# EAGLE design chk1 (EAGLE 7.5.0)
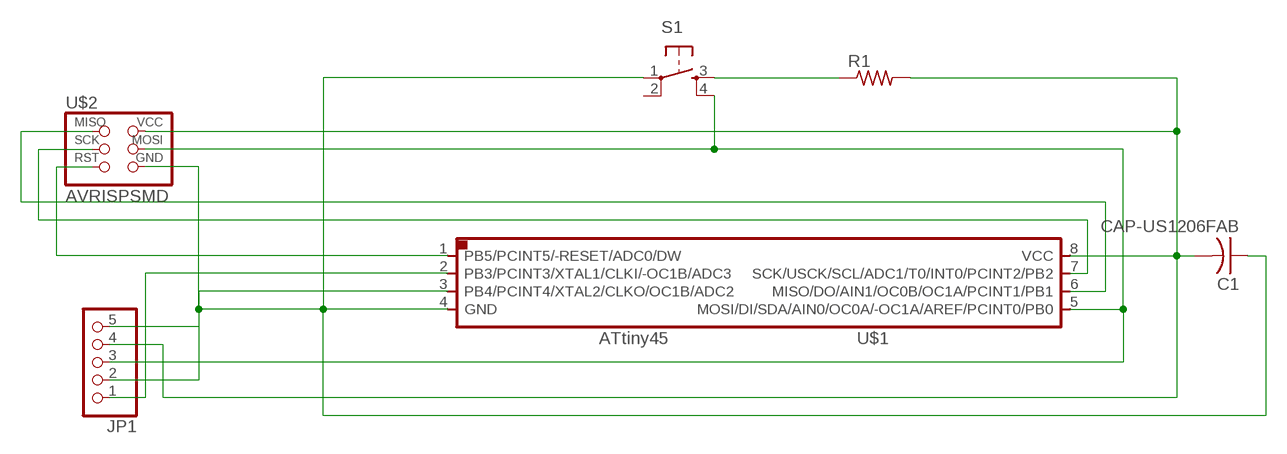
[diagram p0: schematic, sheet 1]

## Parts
C1  CAP-US1206FAB  [C1206FAB]
JP1  PINHD-1X5  [1X05]
R1  RES-US1206FAB  [R1206FAB]
S1  6MM_SWITCH6MM_SWITCH  [6MM_SWITCH]
U$1  ATTINY45SI  [SOIC8]
U$2  AVRISPSMD  [2X03SMD]

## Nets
N$1: C1.1 JP1.5 S1.1(P) U$1.4(GND) U$2.6(GND)
N$2: C1.2 JP1.4 R1.2 U$1.8(VCC) U$2.2(VCC)
N$3: U$1.6(MISO/DO/AIN1/OC0B/OC1A/PCINT1/PB1) U$2.1(MISO)
N$4: U$1.7(SCK/USCK/SCL/ADC1/T0/INT0/PCINT2/PB2) U$2.3(SCK)
N$5: JP1.3 S1.4(S1) U$1.5(MOSI/DI/SDA/AIN0/OC0A/-OC1A/AREF/PCINT0/PB0) U$2.4(MOSI)
N$6: U$1.1(PB5/PCINT5/-RESET/ADC0/DW) U$2.5(RST)
N$7: JP1.2 U$1.3(PB4/PCINT4/XTAL2/CLKO/OC1B/ADC2)
N$8: JP1.1 U$1.2(PB3/PCINT3/XTAL1/CLKI/-OC1B/ADC3)
N$9: R1.1 S1.3(S)
Unconnected: S1.2(P1)

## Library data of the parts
C1 = fab:CAP-US
JP1 = pinhead:PINHD-1X5: PIN HEADER
R1 = fab:RES-US: Resistor (US Symbol)
S1 = fab:6MM_SWITCH: OMRON SWITCH
U$1 = fab:ATTINY45
U$2 = fab:AVRISP

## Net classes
0 default: width 0.406 mm, drill 0.406 mm, clearance 0.406 mm

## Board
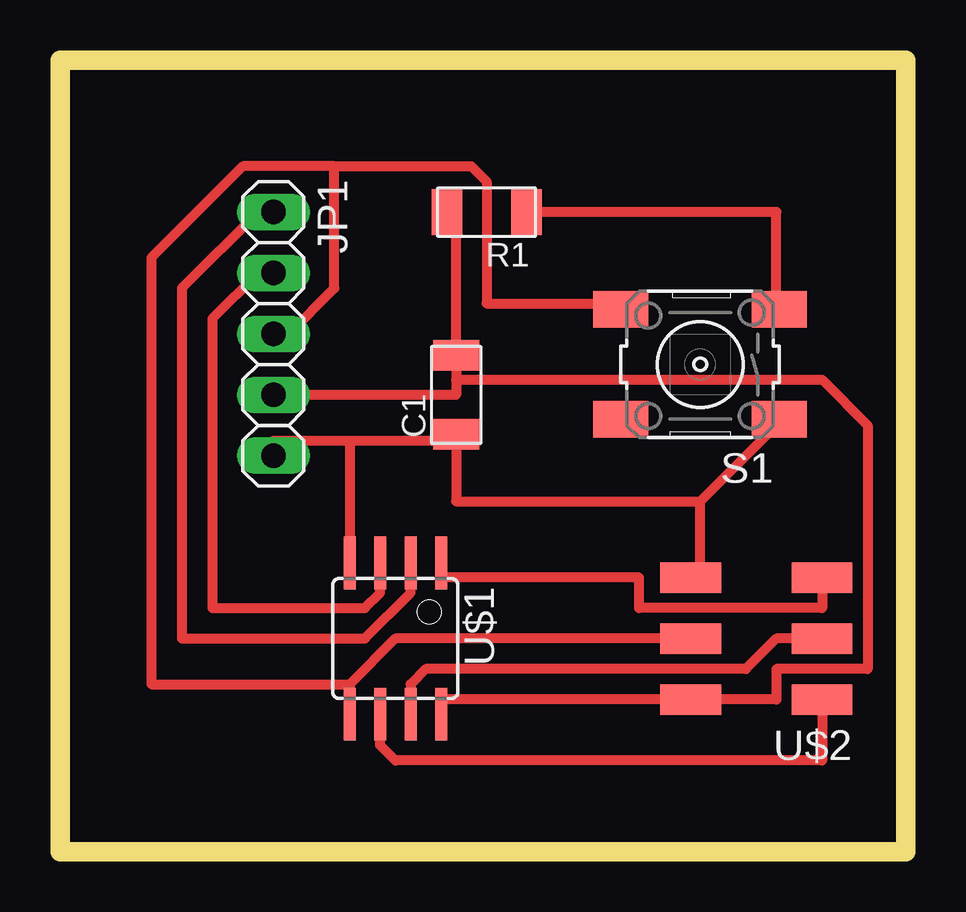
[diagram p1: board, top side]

Size 35.23 x 33.01 mm. Coordinates in mm from the lower left corner, seen from the top.
Outline: 0,0 35.23,0 35.23,33.01 0,33.01 0,0
Copper layers (1*16): Top 0.035mm / dielectric 1.5mm / Bottom 0.035mm
Design rules "default *": minimum track width 10mil, minimum drill 24mil, track to track 17mil, track to pad 17mil, pad to pad 17mil, via to via 17mil, smd to smd 8mil, copper to edge 40mil, drill to drill 8mil, minimum pad ring 10mil, minimum via ring 8mil, stop-mask expansion 4mil, vias tented up to drill 0mil, thermal gap 10mil

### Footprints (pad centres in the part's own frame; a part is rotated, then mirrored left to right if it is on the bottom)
C1206FAB = smd 1.27 x 1.905: 1 -1.651,0; 2 1.651,0
1X05 = drill 1.016 long: 1 -5.08,0; 2 -2.54,0; 3 0,0; 4 2.54,0; 5 5.08,0
R1206FAB = smd 1.27 x 1.905: 1 -1.651,0; 2 1.651,0
6MM_SWITCH = smd 2.286 x 1.524: 1 -3.302,2.286; 2 3.302,2.286; 3 -3.302,-2.286; 4 3.302,-2.286
SOIC8 = smd 0.5 x 2.2: 1 -1.905,-3.154; 2 -0.645,-3.154; 3 0.625,-3.154; 4 1.895,-3.154; 5 1.905,3.154; 6 0.635,3.154; 7 -0.635,3.154; 8 -1.905,3.154
2X03SMD = smd 2.54 x 1.27: 1 -2.54,2.54; 2 2.92,2.54; 3 -2.54,0; 4 2.92,0; 5 -2.54,-2.54; 6 2.92,-2.54

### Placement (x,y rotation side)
C1  16.51,19.05 90 top
JP1  8.89,21.59 270 top
R1  17.78,26.67 180 top
S1  26.67,20.32 180 top
U$1  13.97,8.89 180 top
U$2  29.21,8.89 180 top

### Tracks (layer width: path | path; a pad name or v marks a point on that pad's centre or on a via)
N$1
  Top 0.406: 26.67,14.61 29.85,17.78 S1.1 | 26.67,14.61 26.67,11.43 U$2.6 | 12.06,17.15 8.89,17.15 JP1.5 | 12.06,17.15 16.51,17.15 | 12.06,17.15 12.06,12.07 U$1.4 | 26.67,14.61 16.51,14.61 16.51,17.15 | 16.51,17.15 C1.1
N$2
  Top 0.406: U$1.8 15.88,6.35 U$2.2 29.85,6.35 29.85,7.62 33.66,7.62 33.66,17.78 31.75,19.69 16.51,19.69 | R1.2 16.51,26.67 C1.2 16.51,19.69 | JP1.4 16.51,19.05 16.51,19.69
N$3
  Top 0.406: U$1.6 13.33,4.45 13.97,3.81 31.75,3.81 U$2.1
N$4
  Top 0.406: U$1.7 14.61,6.98 15.24,7.62 28.57,7.62 29.85,8.89 U$2.3
N$5
  Top 0.406: 12.06,6.98 U$1.5 | 12.06,6.98 13.97,8.89 U$2.4 | 11.43,28.58 17.14,28.58 17.78,27.94 17.78,22.86 22.86,22.86 S1.4 | 11.43,28.58 11.43,23.5 9.52,21.59 JP1.3 | 12.06,6.98 3.81,6.98 3.81,24.77 7.62,28.58 11.43,28.58
N$6
  Top 0.406: U$2.5 31.75,10.16 24.13,10.16 24.13,11.43 15.88,11.43 U$1.1
N$7
  Top 0.406: JP1.2 8.25,24.13 6.35,22.23 6.35,10.16 12.7,10.16 13.33,10.8 13.33,11.43 U$1.3
N$8
  Top 0.406: JP1.1 8.25,26.67 5.08,23.5 5.08,8.89 12.7,8.89 14.61,10.8 14.61,11.43 U$1.2
N$9
  Top 0.406: R1.1 29.85,26.67 29.85,22.86 S1.3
